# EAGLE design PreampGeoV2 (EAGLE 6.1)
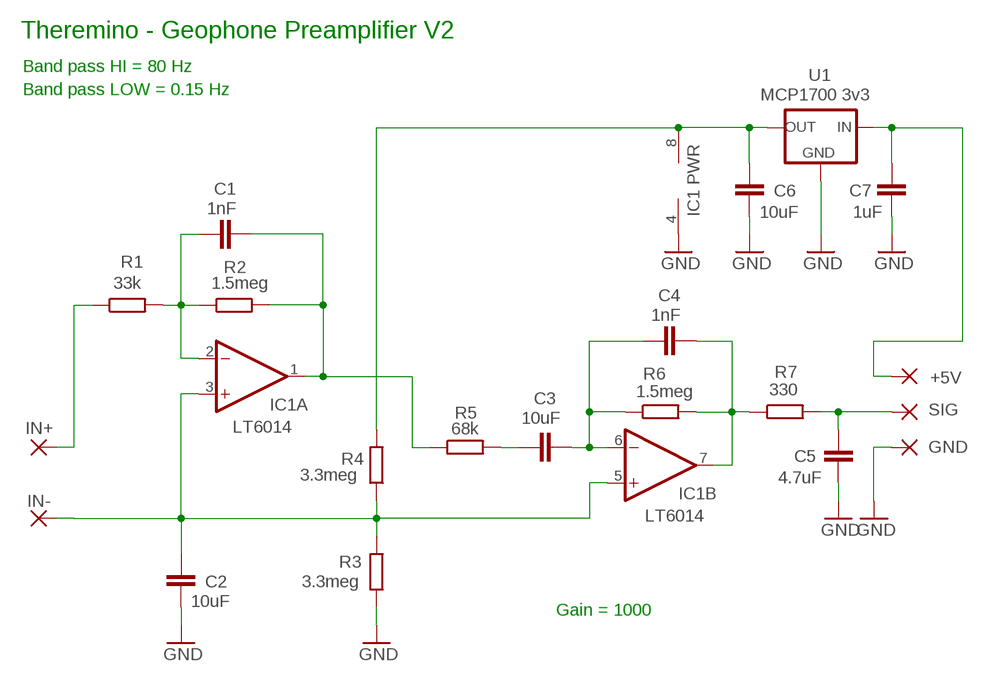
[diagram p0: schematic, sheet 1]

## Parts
+5V  WIREPADSMD1,27-2,54  [SMD1,27-2,54]
C1  1nF  C-EUC0805  [C0805]
C2  10uF  C-EUC0805  [C0805]
C3  10uF  C-EUC0805  [C0805]
C4  1nF  C-EUC0805  [C0805]
C5  4.7uF  C-EUC0805  [C0805]
C6  10uF  C-EUC0805  [C0805]
C7  1uF  C-EUC0805  [C0805]
GND  WIREPADSMD1,27-2,54  [SMD1,27-2,54]
IC1  LT6014  LMC6482D  [SOIC08_S]
IN+  WIREPADSMD1,27-2,54  [SMD1,27-2,54]
IN-  WIREPADSMD1,27-2,54  [SMD1,27-2,54]
R1  33k  R-EU_R0805  [R0805]
R2  1.5meg  R-EU_R0805  [R0805]
R3  3.3meg  R-EU_R0805  [R0805]
R4  3.3meg  R-EU_R1206_L  [R1206_L]
R5  68k  R-EU_R1206_L  [R1206_L]
R6  1.5meg  R-EU_R0805  [R0805]
R7  330  R-EU_R0805  [R0805]
SIG  WIREPADSMD1,27-2,54  [SMD1,27-2,54]
U1  MCP1700 3v3  MCP1700SOT23L  [SOT23_L]

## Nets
GND: C2.2 C5.1 C6.2 C7.2 GND.1(P) IC1.4(P:V-) R3.2 U1.1(GND)
N$1: C1.1 IC1.2(A:-IN) R1.2 R2.1
N$2: C3.1 C4.1 IC1.6(B:-IN) R6.1
N$3: C2.1 IC1.3(A:+IN) IC1.5(B:+IN) IN-.1(P) R3.1 R4.1
N$4: IN+.1(P) R1.1
N$5: C4.2 IC1.7(B:OUT) R6.2 R7.1
N$6: C1.2 IC1.1(A:OUT) R2.2 R5.1
N$7: C5.2 R7.2 SIG.1(P)
N$8: +5V.1(P) C7.1 U1.3(IN)
N$9: C3.2 R5.2
N$12: C6.1 IC1.8(P:V+) R4.2 U1.2(OUT)

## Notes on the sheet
- Theremino - Geophone Preamplifier V2
- Band pass HI = 80 Hz
- Band pass LOW = 0.15 Hz
- IC1 PWR
- Gain = 1000

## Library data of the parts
+5V GND IN+ IN- SIG = 00-LIVIO:WIREPAD: Wire PAD connect wire on PCB
C1-C7 = 00-LIVIO:C-EU: CAPACITOR, European symbol
IC1 = 00-LIVIO:LMC6482: OP AMP
R1-R7 = 00-LIVIO:R-EU_: RESISTOR, European symbol
U1 = 00-LIVIO:MCP1700: Linear regulator Quescient courrent 1.8uA Input 2.3v to 6v Output 1.2v 1.8v 2.5v 3.0v 3.3v 5.0v

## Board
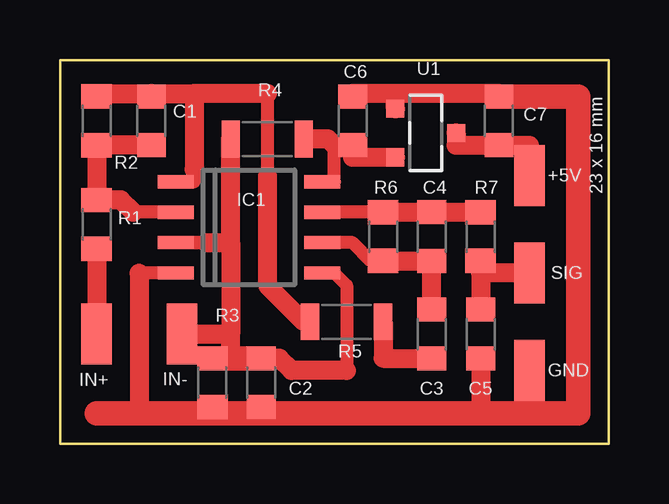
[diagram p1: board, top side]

Size 22.86 x 16 mm. Coordinates in mm from the lower left corner, seen from the top.
Outline: 22.86,0 0,0 0,16 22.86,16 22.86,0
Copper layers (1*16): Top 0.035mm / dielectric 1.5mm / Bottom 0.035mm
Design rules: minimum track width 10mil, minimum drill 28mil, track to track 28mil, track to pad 28mil, pad to pad 28mil, via to via 28mil, smd to smd 28mil, copper to edge 28mil, drill to drill 8mil, minimum pad ring 5mil, minimum via ring 8mil, stop-mask expansion 4mil, vias tented up to drill 0mil, thermal gap 42mil

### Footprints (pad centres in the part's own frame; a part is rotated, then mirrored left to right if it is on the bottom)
SMD1,27-2,54 = smd 1.27 x 2.54: 1 0,0
C0805 = smd 1 x 1.2: 1 -1.016,0; 2 1.016,0
SOIC08_S = smd 0.55 x 1.5: 1 -1.905,-3.048; 2 -0.635,-3.048; 3 0.635,-3.048; 4 1.905,-3.048; 5 1.905,3.048; 6 0.635,3.048; 7 -0.635,3.048; 8 -1.905,3.048
R0805 = smd 1.016 x 1.27: 1 -1.016,0; 2 1.016,0
R1206_L = smd 0.762 x 1.524: 1 -1.524,0; 2 1.524,0
SOT23_L = smd 0.762 x 0.762: 1 -1.016,-1.27; 2 1.016,-1.27; 3 0,1.27

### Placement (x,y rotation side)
+5V  19.56,11.18 0 top
C1  3.81,13.46 90 top
C2  8.38,2.54 270 top
C3  15.49,4.57 270 top
C4  15.49,8.64 90 top
C5  17.53,4.57 90 top
C6  12.19,13.46 90 top
C7  18.29,13.46 90 top
GND  19.56,3.05 0 top
IC1  7.87,9.02 270 top
IN+  1.52,4.57 180 top
IN-  5.08,4.57 0 top
R1  1.52,9.14 90 top
R2  1.52,13.46 90 top
R3  6.35,2.54 270 top
R4  8.64,12.7 0 top
R5  11.94,5.08 0 top
R6  13.46,8.64 90 top
R7  17.53,8.64 270 top
SIG  19.56,7.11 0 top
U1  15.24,12.95 270 top

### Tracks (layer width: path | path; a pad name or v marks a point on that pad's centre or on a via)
GND
  Top 0.55: IC1.4 4.57,7.11 3.3,7.11 | 3.3,1.27 1.52,1.27 | GND.1 19.56,1.27
  Top 0.8: C7.2 18.29,14.61 13.97,14.61 | 13.97,14.61 12.19,14.61 C6.2 | 3.3,7.11 3.3,1.27 | U1.1 13.97,14.61 | C5.1 17.53,1.27
  Top 1.016: 1.52,1.27 3.3,1.27 6.35,1.27 | 6.35,1.27 8.38,1.27 | 8.38,1.27 12.45,1.27 17.53,1.27 19.56,1.27 21.59,1.27 21.59,14.48 C7.2 | R3.2 6.35,1.27 | C2.2 8.38,1.27
N$1
  Top 0.55: IC1.2 3.05,9.65
  Top 0.8: 3.05,9.65 2.54,10.16 R1.2 R2.1 C1.1
N$2
  Top 0.55: R6.1 12.95,7.62 12.19,8.38 IC1.6
  Top 0.8: R6.1 C4.1 C3.1
N$3
  Top 0.55: 7.11,8.38 6.1,8.38 | 6.1,8.38 IC1.3 6.1,8.38 | IC1.5 11.43,7.11 11.94,6.6 11.94,3.05 | R3.1 7.11,3.56
  Top 0.8: 7.11,8.38 R4.1 | 11.94,3.05 9.65,3.05 9.14,3.56 C2.1 | 6.1,8.38 7.11,8.38 | 7.11,8.38 7.11,4.57 | IN-.1 7.11,4.57 | 7.11,3.56 7.11,4.57
  Top 1.016: C2.1 R3.1
N$4
  Top 0.8: R1.1 IN+.1
N$5
  Top 0.55: R6.2 IC1.7
  Top 0.8: R6.2 C4.2 R7.1
N$6
  Top 0.55: IC1.1 5.59,10.92 5.59,11.43 | 8.64,14.61 8.64,11.18
  Top 0.8: 8.64,11.18 8.64,6.6 10.16,5.08 R5.1 | R2.2 1.52,14.61 3.81,14.61 | 3.81,14.61 C1.2 3.81,14.61 | 3.81,14.61 5.59,14.61 | 5.59,14.61 5.59,11.43 | 8.64,14.61 5.84,14.61 5.59,14.61
N$7
  Top 0.55: R7.2 17.53,7.11 R7.2
  Top 0.8: C5.2 17.53,7.11 SIG.1
N$8
  Top 0.8: +5V.1 19.56,12.45 C7.1 16.51,12.45 U1.3
N$9
  Top 0.8: R5.2 13.46,3.56 C3.2
N$12
  Top 0.55: IC1.8 11.43,10.92 11.43,12.45
  Top 0.8: R4.2 11.18,12.7 11.43,12.45 C6.1 12.19,11.94 U1.2

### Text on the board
tNames: 23 x 16 mm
